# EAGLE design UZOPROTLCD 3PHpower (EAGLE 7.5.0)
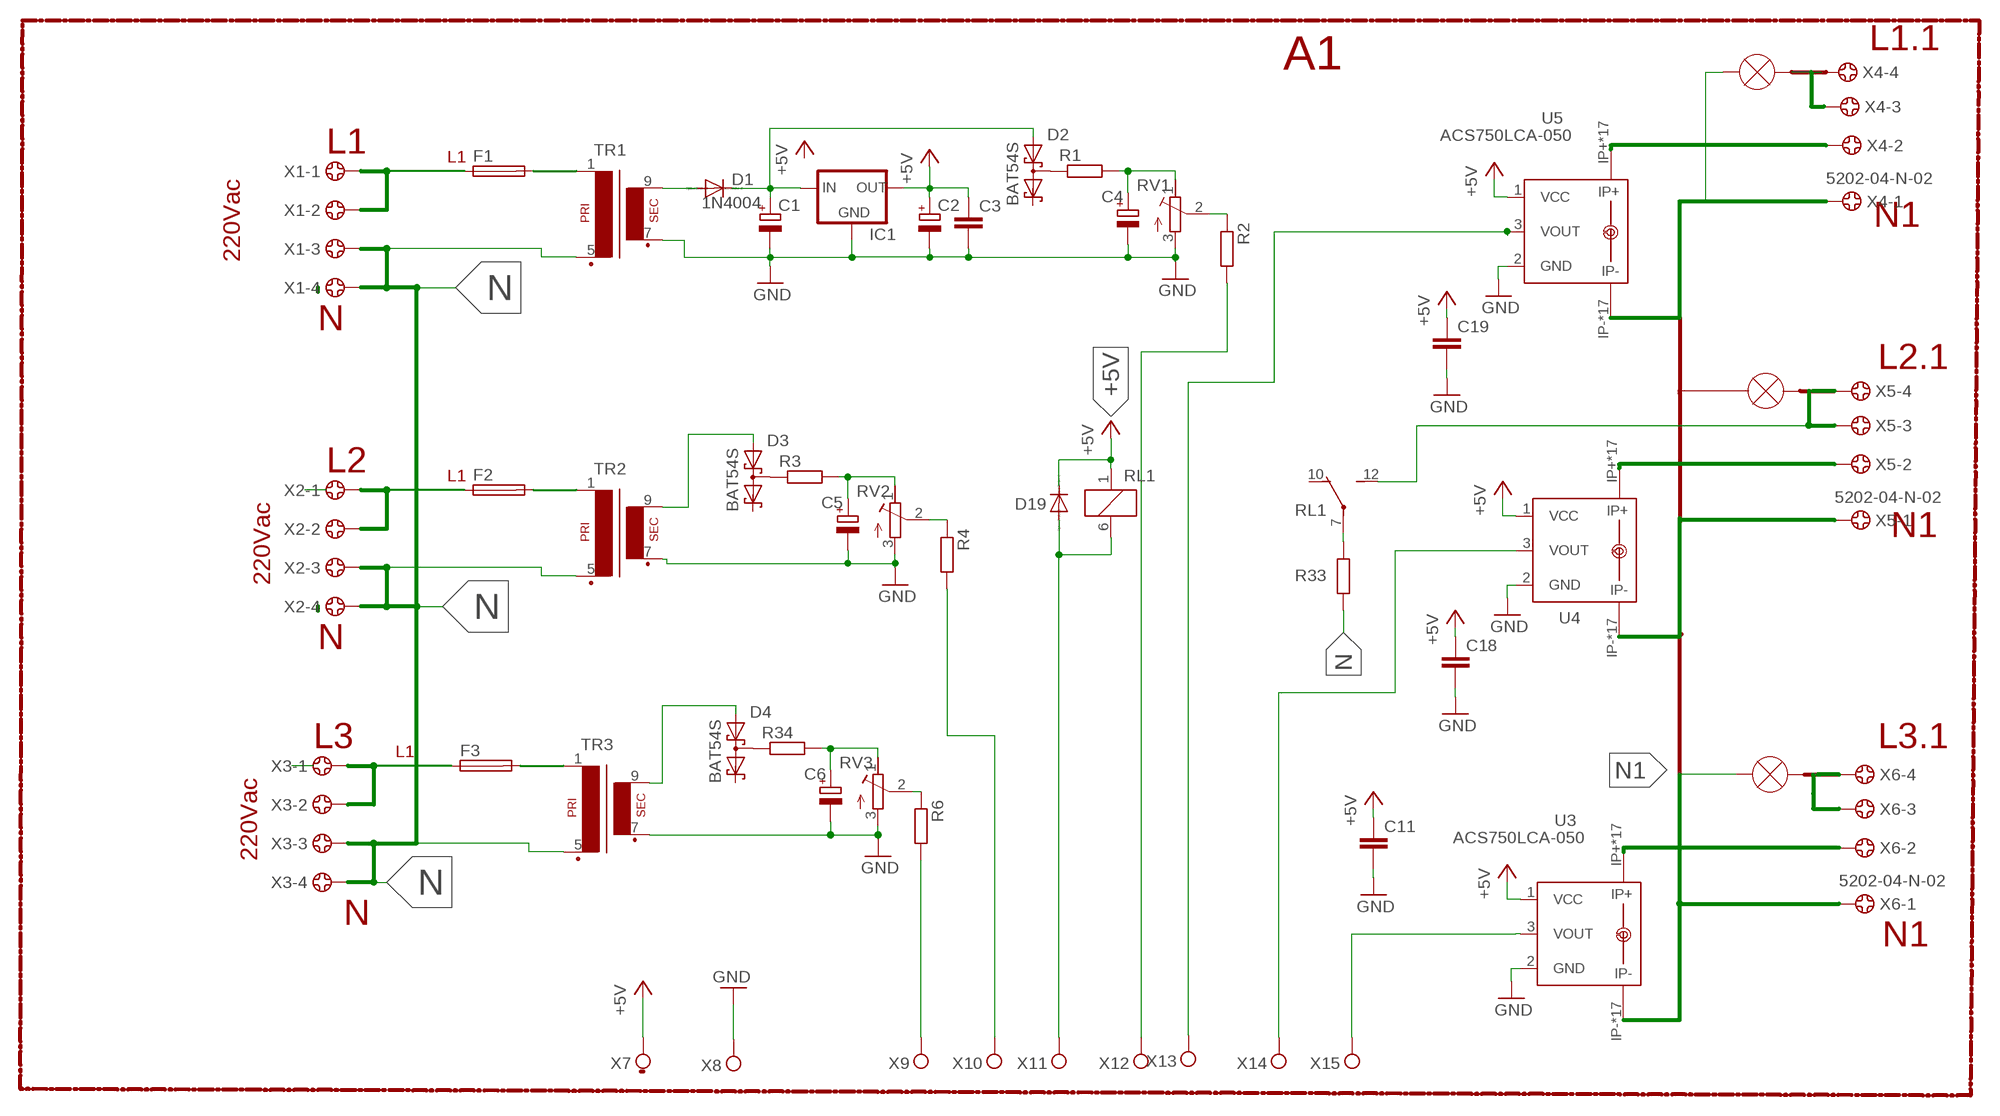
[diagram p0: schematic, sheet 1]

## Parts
C1  CPOL-EUE5-10.5  [E5-10,5]
C2  CPOL-EUE2-5  [E2-5]
C3  C-EUC1206  [C1206]
C4  CPOL-EUE2-5  [E2-5]
C5  CPOL-EUE2-5  [E2-5]
C6  CPOL-EUE2-5  [E2-5]
C11  C-EUC1206  [C1206]
C18  C-EUC1206  [C1206]
C19  C-EUC1206  [C1206]
D1  1N4004  [DO41-10]
D2  BAT54S  [SOT23]
D3  BAT54S  [SOT23]
D4  BAT54S  [SOT23]
D19  1N4148DO35-7  [DO35-7]
F1  FUSEGSH15 1A 5x20mm  FUSEGSH15  [GSH15]
F2  FUSEGSH15 1A 5x20mm  FUSEGSH15  [GSH15]
F3  FUSEGSH15 1A 5x20mm  FUSEGSH15  [GSH15]
IC1  78XXL  [78XXL]
R1  R-EU_R1206  [R1206]
R2  R-EU_R1206  [R1206]
R3  R-EU_R1206  [R1206]
R4  R-EU_R1206  [R1206]
R6  R-EU_R1206  [R1206]
R33  R-EU_0617/5V  [0617V]
R34  R-EU_R1206  [R1206]
RL1  G6E-134  [G6E]
RV1  R-TRIMM-3386-F  [R-TRIMM-3386F]
RV2  R-TRIMM-3386-F  [R-TRIMM-3386F]
RV3  R-TRIMM-3386-F  [R-TRIMM-3386F]
TR1  EI42-1  [EI42-1]
TR2  EI42-1  [EI42-1]
TR3  EI42-1  [EI42-1]
U3  ACS750LCA-050  [ACS75050]
U4  ACS750LCA-050  [ACS75050]
U5  ACS750LCA-050  [ACS75050]
X1  5202-04-N-02  [5202-04-N-02]
X2  5202-04-N-02  [5202-04-N-02]
X3  5202-04-N-02  [5202-04-N-02]
X4  5202-04-N-02  [5202-04-N-02]
X5  5202-04-N-02  [5202-04-N-02]
X6  5202-04-N-02  [5202-04-N-02]
X7  TPPAD1-17  [P1-17]
X8  TPPAD1-17  [P1-17]
X9  TPPAD1-17  [P1-17]
X10  TPPAD1-17  [P1-17]
X11  TPPAD1-17  [P1-17]
X12  TPPAD1-17  [P1-17]
X13  TPPAD1-17  [P1-17]
X14  TPPAD1-17  [P1-17]
X15  TPPAD1-17  [P1-17]

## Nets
+5V: C2.+ C3.1 C11.1 C18.1 C19.1 D19.C IC1.OUT RL1.1 U3.1(VCC) U4.1(VCC) U5.1(VCC) X7.TP
GND: C1.- C2.- C3.2 C4.- C5.- C6.- C11.2 C18.2 C19.2 IC1.GND RV1.3(E) RV2.3(E) RV3.3(E) TR1.7(S3) TR2.7(S3) TR3.7(S3) U3.2(GND) U4.2(GND) U5.2(GND) X8.TP
N: R33.1 TR1.5(P2) TR2.5(P2) TR3.5(P2) X1.3 X1.4 X2.3 X2.4 X3.3 X3.4
N1: U3.IP- U3.IP-@2(IP-) U3.IP-@3(IP-) U3.IP-@4(IP-) U3.IP-@5(IP-) U3.IP-@6(IP-) U3.IP-@7(IP-) U3.IP-@8(IP-) U3.IP-@9(IP-) U3.IP-@10(IP-) U3.IP-@11(IP-) U3.IP-@12(IP-) U3.IP-@13(IP-) U3.IP-@14(IP-) U3.IP-@15(IP-) U3.IP-@16(IP-) U3.IP-@17(IP-) X6.1
N$1: U5.IP- U5.IP-@2(IP-) U5.IP-@3(IP-) U5.IP-@4(IP-) U5.IP-@5(IP-) U5.IP-@6(IP-) U5.IP-@7(IP-) U5.IP-@8(IP-) U5.IP-@9(IP-) U5.IP-@10(IP-) U5.IP-@11(IP-) U5.IP-@12(IP-) U5.IP-@13(IP-) U5.IP-@14(IP-) U5.IP-@15(IP-) U5.IP-@16(IP-) U5.IP-@17(IP-) X4.1
N$2: D2.3(C1A2) R1.1
N$3: F2.1 X2.1 X2.2
N$4: F2.2 TR2.1
N$5: D19.A RL1.6 X11.TP
N$7: F3.1 X3.1 X3.2
N$8: F3.2 TR3.1
N$9: F1.1 X1.1 X1.2
N$10: F1.2 TR1.1
N$11: U4.IP- U4.IP-@2(IP-) U4.IP-@3(IP-) U4.IP-@4(IP-) U4.IP-@5(IP-) U4.IP-@6(IP-) U4.IP-@7(IP-) U4.IP-@8(IP-) U4.IP-@9(IP-) U4.IP-@10(IP-) U4.IP-@11(IP-) U4.IP-@12(IP-) U4.IP-@13(IP-) U4.IP-@14(IP-) U4.IP-@15(IP-) U4.IP-@16(IP-) U4.IP-@17(IP-) X5.1
N$12: RL1.12(S) X5.3 X5.4
N$13: D1.A TR1.9(S4)
N$14: C4.+ R1.2 RV1.1(A)
N$15: C1.+ D1.C D2.1(A1) IC1.IN
N$16: X4.3 X4.4
N$17: D3.1(A1) TR2.9(S4)
N$19: R2.1 RV1.2(S)
N$20: D3.3(C1A2) R3.1
N$21: C5.+ R3.2 RV2.1(A)
N$22: R4.1 RV2.2(S)
N$23: U5.IP+ U5.IP+@2(IP+) U5.IP+@3(IP+) U5.IP+@4(IP+) U5.IP+@5(IP+) U5.IP+@6(IP+) U5.IP+@7(IP+) U5.IP+@8(IP+) U5.IP+@9(IP+) U5.IP+@10(IP+) U5.IP+@11(IP+) U5.IP+@12(IP+) U5.IP+@13(IP+) U5.IP+@14(IP+) U5.IP+@15(IP+) U5.IP+@16(IP+) U5.IP+@17(IP+) X4.2
N$24: U4.IP+ U4.IP+@2(IP+) U4.IP+@3(IP+) U4.IP+@4(IP+) U4.IP+@5(IP+) U4.IP+@6(IP+) U4.IP+@7(IP+) U4.IP+@8(IP+) U4.IP+@9(IP+) U4.IP+@10(IP+) U4.IP+@11(IP+) U4.IP+@12(IP+) U4.IP+@13(IP+) U4.IP+@14(IP+) U4.IP+@15(IP+) U4.IP+@16(IP+) U4.IP+@17(IP+) X5.2
N$25: D4.1(A1) TR3.9(S4)
N$26: D4.3(C1A2) R34.1
N$27: C6.+ R34.2 RV3.1(A)
N$28: R6.1 RV3.2(S)
N$29: R33.2 RL1.7(P)
N$30: X6.3 X6.4
N$32: U3.IP+ U3.IP+@2(IP+) U3.IP+@3(IP+) U3.IP+@4(IP+) U3.IP+@5(IP+) U3.IP+@6(IP+) U3.IP+@7(IP+) U3.IP+@8(IP+) U3.IP+@9(IP+) U3.IP+@10(IP+) U3.IP+@11(IP+) U3.IP+@12(IP+) U3.IP+@13(IP+) U3.IP+@14(IP+) U3.IP+@15(IP+) U3.IP+@16(IP+) U3.IP+@17(IP+) X6.2
N$33: R6.2 X9.TP
N$34: R4.2 X10.TP
N$36: R2.2 X12.TP
N$37: U5.3(VOUT) X13.TP
N$38: U4.3(VOUT) X14.TP
N$39: U3.3(VOUT) X15.TP
Unconnected: D2.2(C2) D3.2(C2) D4.2(C2) RL1.10(O)

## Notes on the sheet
- L1.1
- A1
- L1
- L1
- N1
- 220Vac
- N
- L2.1
- L2
- L1
- N1
- 220Vac
- N
- L3 | L3.1
- L1
- 220Vac
- N
- N1

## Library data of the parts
C1 C2 C4-C6 = rcl:CPOL-EU: POLARIZED CAPACITOR, European symbol
C3 C11 C18 C19 = rcl:C-EU: CAPACITOR, European symbol
D1 = diode:1N4004: DIODE
D2-D4 = diode:BAT54S: Schottky Diodes Pin connection corrected 2011-05-04 Source: Fairchild .. BAT54.pdf
D19 = diode:1N4148: DIODE
F1-F3 = fuse:FUSE: Fuse; OC_FARNELL: unknown; OC_NEWARK: unknown
IC1 = v-reg:78XXL: VOLTAGE REGULATOR
R1-R4 R6 R33 R34 = rcl:R-EU_: RESISTOR, European symbol
RL1 = relay:G6E-134
RV1-RV3 = rcl:R-TRIMM-3386-F
TR1-TR3 = trafo:EI42-1: TRANSFORMER 1 primary winding, 1 secondary winding ERA
U3-U5 = allegro:ACS750*CA-050: Current Sensor display layer 49 Reference in BRD and place VIAs on circles Source: www.allegromicro.com/datafile/0750-050.pdf; MF: ALLEGRO MICROSYSTEMS, INC.; MPN: ACS750LCA-050; OC_FARNELL: 1457176; OC_NEWARK: 61H4464
X1-X6 = con-ebyelectro:5202-04-N-02: Barrier Blocks Sreies 5202 Source: http://www.ebyelectro.com/PDF/5202-XX-N-02.pdf; OC_FARNELL: unknown; OC_NEWARK: unknown
X7-X15 = testpad:TP: Test pad

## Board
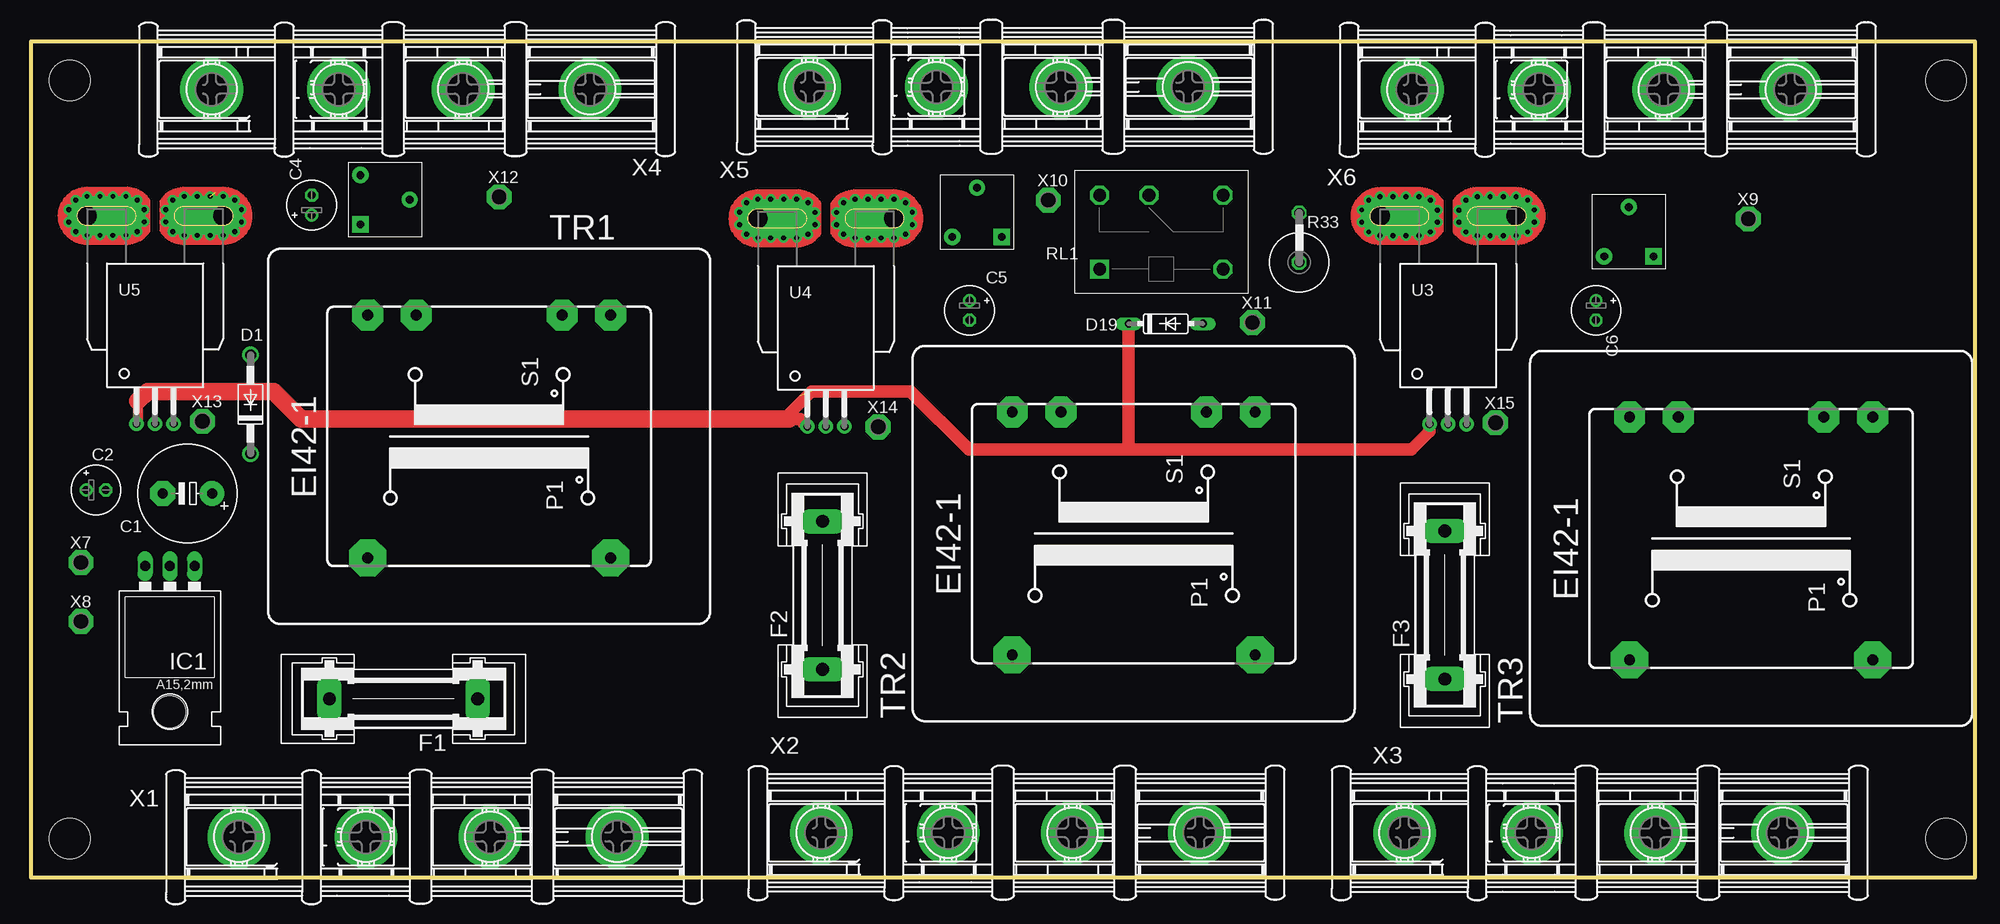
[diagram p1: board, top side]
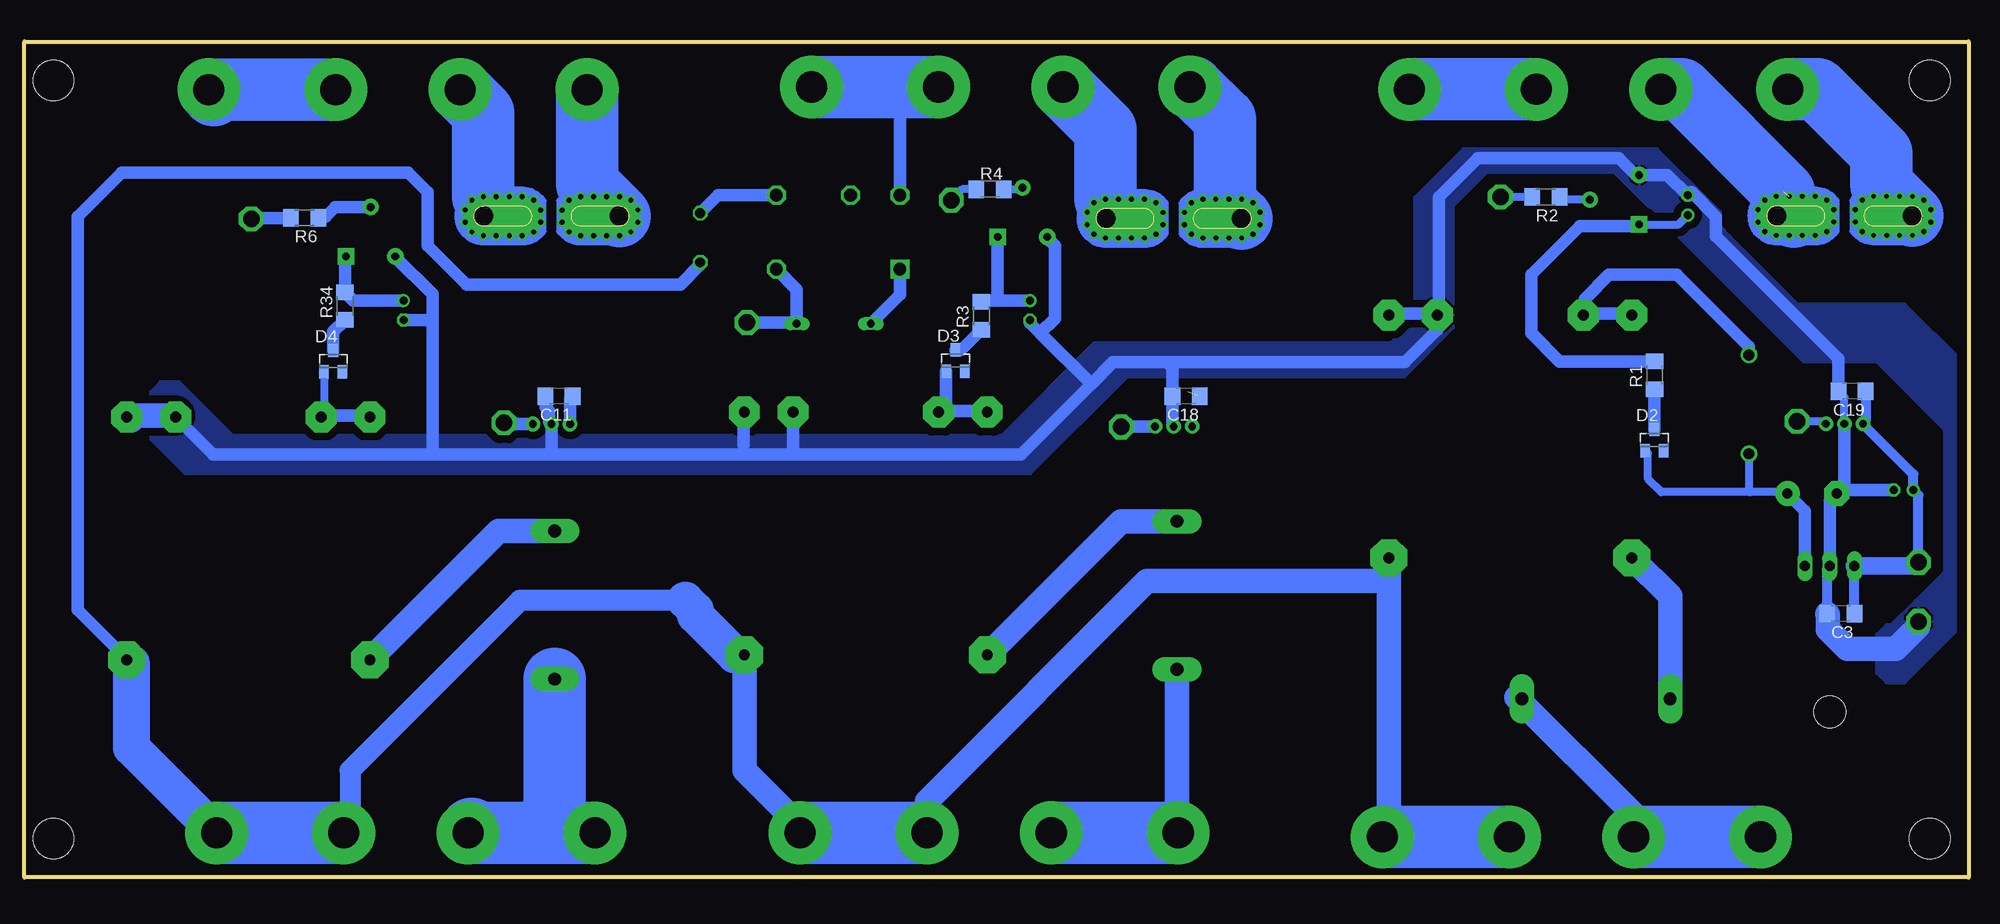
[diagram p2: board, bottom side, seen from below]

Size 200 x 86 mm. Coordinates in mm from the lower left corner, seen from the top.
Outline: 200,0 200,86 0,86 0,0 200,0
Copper layers (1*16): Top 0.035mm / dielectric 1.5mm / Bottom 0.035mm
Design rules "default": minimum track width 10mil, minimum drill 24mil, track to track 8mil, track to pad 8mil, pad to pad 8mil, via to via 8mil, smd to smd 8mil, copper to edge 40mil, drill to drill 8mil, minimum pad ring 10mil, minimum via ring 8mil, stop-mask expansion 4mil, vias tented up to drill 0mil, thermal gap 10mil
Holes 4.2 mm at 4,82 4,4 197,4 197,82

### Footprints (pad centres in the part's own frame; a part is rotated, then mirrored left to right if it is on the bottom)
E5-10,5 = drill 1.016 pad 2.54: + -2.54,0 | drill 1.016 pad 2.54 octagon: - 2.54,0
E2-5 = drill 0.813 pad 1.27: + -1.016,0 | drill 0.813 pad 1.27 octagon: - 1.016,0
C1206 = smd 1.6 x 1.8: 1 -1.4,0; 2 1.4,0
DO41-10 = drill 1.118: A 5.08,0; C -5.08,0
SOT23 = smd 1 x 1.4: 1 -0.95,-1.1; 2 0.95,-1.1; 3 0,1.1
DO35-7 = drill 0.813 long: A 3.81,0; C -3.81,0
GSH15 = drill 1.321 pad 2.54 long: 1 -7.62,0; 2 7.62,0
78XXL = drill 1.016 long: GND 0,-3.81; IN -2.54,-3.81; OUT 2.54,-3.81 | hole 3.302: 0,11.176
R1206 = smd 1.6 x 1.803: 1 -1.422,0; 2 1.422,0
0617V = drill 1.016 octagon: 1 -2.54,0; 2 2.54,0
G6E = drill 1.3 square: 1 0,0 | drill 1.3 octagon: 6 12.7,0; 7 12.7,7.62; 10 5.08,7.62; 12 0,7.62
R-TRIMM-3386F = drill 0.8 pad 1.676 square: 1 0,0 | drill 0.8 pad 1.676: 2 5.08,2.54; 3 0,5.08
EI42-1 = drill 1.118 pad 3.81 octagon: 1 -12.497,12.497; 5 -12.497,-12.497 | drill 1.118 pad 3.175 octagon: 6 12.497,-12.497; 7 12.497,-7.493; 9 12.497,7.493; 10 12.497,12.497
ACS75050 = drill 0.8 pad 1.5: 1 -1.91,-21.4; 2 0,-21.4; 3 1.91,-21.4 | drill 2 pad 4 offset: IP+ 7,0; IP- -7,0 | drill 0.5 pad 0.9: IP+@2 8.89,-0.635; IP+@3 8.89,0.635; IP+@4 8.175,1.625; IP+@5 7,2; IP+@6 5.675,2; IP+@7 4.325,2; IP+@8 3,2; IP+@9 1.825,1.625; IP+@10 1.1,0.625; IP+@11 1.1,-0.625; IP+@12 1.825,-1.625; IP+@13 3,-2; IP+@14 4.325,-2; IP+@15 5.675,-2; IP+@16 7,-2; IP+@17 8.175,-1.625; IP-@2 -8.89,-0.635; IP-@3 -8.89,0.635; IP-@4 -8.175,1.625; IP-@5 -7,2; IP-@6 -5.675,2; IP-@7 -4.325,2; IP-@8 -3,2; IP-@9 -1.825,1.625; IP-@10 -1.1,0.625; IP-@11 -1.1,-0.625; IP-@12 -1.825,-1.625; IP-@13 -3,-2; IP-@14 -4.35,-2; IP-@15 -5.675,-2; IP-@16 -7,-2; IP-@17 -8.175,-1.625
5202-04-N-02 = drill 3.2 pad 6.452: 1 -14.875,0; 2 -1.815,0; 3 10.975,0; 4 24.035,0
P1-17 = drill 1.702 pad 2.54 octagon: TP 0,0

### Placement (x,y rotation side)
C1  16.1,39.49 180 top
C2  6.7,39.85 0 top
C3  13.16,27.12 180 bottom
C4  28.9,69.16 90 top
C5  96.55,58.34 270 top
C6  161,58.34 270 top
C11  145,49.5 180 bottom
C18  80.5,49.5 180 bottom
C19  12,50 180 bottom
D1  22.6,48.67 90 top
D2  32.34,45 0 bottom
D3  104.22,53.17 0 bottom
D4  168.22,53.12 0 bottom
D19  116.74,56.96 0 top
F1  38.33,18.37 180 top
F2  81.43,29.02 90 top
F3  145.44,28.02 90 top
IC1  14.3,28.22 180 top
R1  32.3,51.66 90 bottom
R2  43.5,70 180 bottom
R3  101.55,57.78 90 bottom
R4  100.66,70.8 180 bottom
R6  171.16,67.85 180 bottom
R33  130.47,65.82 90 top
R34  167,58.78 90 bottom
RL1  109.93,62.58 0 top
RV1  33.89,67.18 0 top
RV2  99.87,65.89 90 top
RV3  166.92,63.89 90 top
TR1  47.14,45.37 90 top
TR2  113.44,35.37 90 top
TR3  176.95,34.87 90 top
U3  145.78,68.04 0 top
U4  81.78,67.8 0 top
U5  12.78,68.06 0 top
X1  36.28,4.16 0 top
X2  96.18,4.58 0 top
X3  156.18,4.57 0 top
X4  33.48,81.08 0 top
X5  94.98,81.32 0 top
X6  156.98,81.06 0 top
X7  5.16,32.41 0 top
X8  5.16,26.33 0 top
X9  176.66,67.75 0 top
X10  104.66,69.67 0 top
X11  125.66,57.09 0 top
X12  48.16,70.01 0 top
X13  17.66,46.93 0 top
X14  87.16,46.35 0 top
X15  150.66,46.77 0 top

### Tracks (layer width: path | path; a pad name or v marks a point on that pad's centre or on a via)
+5V  (1 unrouted)
  Top 1.016: 11,49 11,46.79 U5.1
  Top 1.27: 79.5,46.77 U4.1 79.1,47.17 78,47.17 | U3.1 143.87,45.87 142,44 113,44 | 113,44 96.5,44 90.5,50 80.33,50 77.5,47.17 | D19.C 112.93,44.07 113,44
  Top 1.778: 78,47.17 77.5,47.17 27.83,47.17 25,50 12,50 11,49
  Bottom 1.016: X7.TP 5.16,39.33 C2.+ 5.68,41.47 U5.1 10.6,46.93 C19.1 | C3.1 IC1.OUT
  Bottom 1.27: RL1.1 109.93,59.96 D19.C | C11.1 143.87,49.23 U3.1
  Bottom 1.778: IC1.OUT 5.54,32.03 X7.TP
GND
  Bottom 0.813: U5.2 12.78,49.38 C19.2
  Bottom 1.016: C3.2 14.56,31.77 IC1.GND
  Bottom 1.27: C19.2 13.4,53.4 26,66 26,68 28.5,70.5 28.58,70.5 C4.- 30.98,72.26 RV1.3 34.26,72.26 36,74 50.5,74 54.5,70 54.5,58 TR1.7 54.63,56.37 58,53 82.5,53 | 82.5,53 88,53 90.25,50.75 | 90.25,50.75 97.5,43.5 120.5,43.5 | 120.5,43.5 146,43.5 | 146,43.5 158,43.5 | 158,43.5 180.58,43.5 TR3.7 | TR2.7 120.93,43.93 120.5,43.5 | U4.2 81.9,46.52 C18.2 81.9,52.4 82.5,53 | C5.- 96.55,57.05 95.5,56 | 95.5,56 90.25,50.75 | RV2.3 94.79,65.79 94,65 94,57.5 95.5,56 | IC1.GND 14.3,38.75 C1.- | U5.2 12.78,40.27 C1.- | C2.- 13.2,39.85 C1.- | 146,43.5 145.78,43.72 U3.2 146,46.86 146,48 146.4,48.4 C11.2 | 158,57.5 158.18,57.32 C6.- | 158,57.5 158,43.5 | RV3.3 161.84,63.84 158,60 158,57.5 | 126,48 126,44.5
  Bottom 2.54: X8.TP 5.16,25.84 7.5,23.5 12.5,23.5 14.5,25.5 14.5,27.06 C3.2
  pour Bottom (isolate 0.813): 8.5,26 8,26 5.5,28.5 2.5,31.5 2.5,46 9.5,53 17,53 36.5,72.5 49.5,72.5 53,69 53,56.5 58,51.5 86.5,51.5 96.5,41.5 183.5,41.5 187,45 187,50 186,51 184,51 178.5,45.5 99.5,45.5 90,55 59.5,55 57,57.5 57,70 52,75 32,75 25.5,68.5 25.5,67 24.5,66 17.5,59 6.5,59 0.5,53 0.5,26 6.5,20 8.5,20 9.5,21 9.5,25
N
  Bottom 1.27: R33.1 130.47,63.03 132.5,61 154.5,61 158.5,65 158.5,70.5 160.5,72.5 190,72.5 194.5,68 194.5,27.5 189,22 189.07,22 TR3.5
  Bottom 2.184: 132,28.5 149,28.5 166.5,11 166.5,5.22 X3.3
  Bottom 2.54: TR2.5 125.94,11.02 119.5,4.58 | TR1.5 59.64,30.5 | 59.64,30.5 59.64,4.84 X1.4 | X2.3 107.16,7.84 84.5,30.5 59.64,30.5
  Bottom 3.81: 189,22 189,13.36 X3.4 | TR2.5 126.87,22.87 131,27 131,27.5 132,28.5
  Bottom 6.452: X3.3 X3.4 | X2.4 119.5,4.58 X2.3 | X1.3 X1.4
N1
  Bottom 6.452: X6.1 142.1,71.36 U3.IP-
N$1
  Bottom 6.452: X4.1 15.58,81.08 9,74.5 9,71.28 U5.IP-
N$2
  Bottom 1.27: D2.3 32.34,50.2 R1.1
N$3
  Bottom 2.54: F2.1 81.43,4.71 X2.1
  Bottom 6.452: X2.1 X2.2
N$4
  Bottom 2.54: F2.2 87.18,36.64 TR2.1
N$5
  Bottom 1.27: RL1.6 120.55,60.5 D19.A 120.68,57.09 X11.TP
N$6
  Bottom 1.27: 35,58 39.5,58
N$7
  Bottom 6.452: X3.1 147,4.57 | 147,4.57 153.57,4.57 154,5 154,4.93 X3.2 | F3.1 145.44,6.13 147,4.57
N$8
  Bottom 2.54: F3.2 151.19,35.64 TR3.1
N$9
  Bottom 2.54: X1.2 34.47,6.46 46.5,18.5 46.08,18.5 F1.1
  Bottom 6.452: X1.1 X1.2
N$10
  Bottom 2.54: F1.2 30.71,28.94 TR1.1
N$11
  Bottom 6.452: X5.1 79.82,81.32 76.5,78 76.5,69.52 U4.IP-
N$12
  Bottom 1.27: RL1.12 109.93,80.89 109.5,81.32
  Bottom 6.452: X5.3 109.5,81.32 X5.4
N$13
  Bottom 1.27: D1.A 22.6,54.6 30,62 37,62 39.5,59.5 39.5,58.01 TR1.9
N$14
  Bottom 0.813: RV1.1 29.86,67.18 C4.+
  Bottom 1.27: R1.2 42.08,53.08 45,56 45,62 40,67 34.07,67 RV1.1
N$15
  Bottom 0.813: 18.64,39.63 22.5,39.63 | 22.5,39.63 31.63,39.63 33,41 33,43.61 D2.1 | D1.C 22.6,39.73 22.5,39.63
  Bottom 1.27: IC1.IN 16.84,37.69 C1.+ 18.64,39.63
N$16
  Bottom 6.452: X4.4 X4.3
N$17
  Bottom 1.27: D3.1 105.17,48.64 TR2.9
N$18
  Bottom 1.27: 59.5,58 55,58
N$19
  Bottom 0.813: RV1.2 41.8,69.72 R2.1
N$20
  Bottom 1.27: D3.3 103.64,54.27 R3.1
N$21
  Bottom 1.27: C5.+ 100,59.36 | 100,59.36 101.4,59.36 R3.2 | RV2.1 99.87,59.49 100,59.36
N$22
  Bottom 0.813: R4.1 97.5,70.8 RV2.2
N$23  (1 unrouted)
  Bottom 6.452: X4.2 29.58,81.08 19,70.5 19,69 18,68
N$24
  Bottom 6.452: U4.IP+@5 88.78,76.94 X5.2
N$25
  Bottom 0.813: D4.1 169.17,47.65 TR3.9
N$26
  Bottom 1.27: D4.3 168.22,56.14 R34.1
N$27
  Bottom 1.27: C6.+ 166.15,59.36 R34.2 167,63.81 RV3.1
N$28
  Bottom 1.27: RV3.2 168.03,68.97 169,68 169.59,68 R6.1
N$29
  Bottom 1.27: RL1.7 128.63,70.2 R33.2
N$30
  Bottom 6.452: X6.3 179.94,81.06 180.5,80.5 180.5,80.55 X6.4
N$31
  Bottom 1.27: 101,48 105.5,48 106,47.5
N$32
  Bottom 6.452: U3.IP+@5 152.78,78.67 X6.2
N$33
  Bottom 1.27: R6.2 176.56,67.85 X9.TP
N$34
  Bottom 0.813: R4.2 103.53,70.8 X10.TP
N$35
  Bottom 2.54: 189,47.5 188.5,47.5 | 184.5,47.5 188.5,47.5 | 188.5,47.5 189,47 189.5,47.5
N$36
  Bottom 0.813: R2.2 X12.TP
N$37
  Bottom 0.813: X13.TP 14.96,46.93 U5.3
N$38
  Bottom 1.27: U4.3 87.11,46.4 X14.TP
N$39
  Bottom 1.27: U3.3 150.53,46.64 X15.TP
N$40
  Bottom 1.27: 164.5,47.5 169.5,47.5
